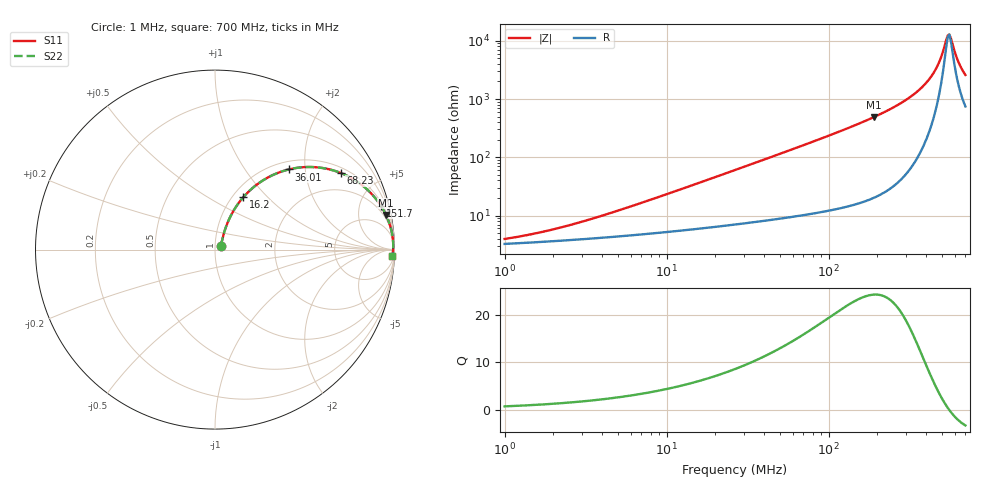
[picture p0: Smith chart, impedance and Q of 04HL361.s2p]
! Coilcraft 0402HL-361 Chip Inductor
! 20 July 2012
# MHz S MA R 50
!Freq  MagS11  AngS11  MagS21  AngS21  MagS12  AngS12  MagS22  AngS22
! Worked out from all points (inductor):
!   288 points, 1 MHz to 700 MHz, reference 50 ohm
!   read as one part in series: L = 360 nH near 6.21 MHz
!   highest Q = 24.2 at 190.6 MHz (marker M1), where L = 408 nH
!   self-resonance near 544.6 MHz
!   S11 on the Smith chart (normalised r, x): 1 MHz: 1.07, +0.05; 16.2 MHz: 1.12, +0.73; 36.01 MHz: 1.16, +1.64; 68.23 MHz: 1.20, +3.13; 151.7 MHz: 1.32, +7.42; 700 MHz: 16, -50
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1  0.03842 33.5  0.9682 -1.3  0.9682 -1.3  0.03842 33.5
1.690458  0.05023 45.2  0.9652 -2.1  0.9652 -2.1  0.05023 45.2
2.991129  0.07507 56.2  0.9603 -3.7  0.9603 -3.7  0.07507 56.2
8.946856  0.195 65.1  0.9347 -10.9  0.9347 -10.9  0.195 65.1
16.19625  0.3313 61.6  0.8917 -19.1  0.8917 -19.1  0.3313 61.6
26.7612  0.4964 53.8  0.8128 -29.5  0.8128 -29.5  0.4964 53.8
36.00623  0.6072 47.4  0.739 -37.2  0.739 -37.2  0.6072 47.4
49.56361  0.7226 39.5  0.6374 -46.1  0.6374 -46.1  0.7226 39.5
68.22573  0.82 31.4  0.5222 -54.9  0.5222 -54.9  0.82 31.4
80.04622  0.8593 27.6  0.4639 -59.1  0.4639 -59.1  0.8593 27.6
151.6741  0.9553 14.9  0.2573 -72.6  0.2573 -72.6  0.9553 14.9
190.5653  0.9719 11.4  0.1986 -76.2  0.1986 -76.2  0.9719 11.4
239.4286  0.9827 8.5  0.1475 -79.1  0.1475 -79.1  0.9827 8.5
329.5804  0.991 4.9  0.08592 -81.5  0.08592 -81.5  0.991 4.9
414.089  0.9932 2.7  0.04711 -80.4  0.04711 -80.4  0.9932 2.7
474.8682  0.9933 1.4  0.0254 -74.1  0.0254 -74.1  0.9933 1.4
508.5255  0.993 0.8  0.01534 -62.6  0.01534 -62.6  0.993 0.8
544.5684  0.9925 0.2  0.008032 -21.2  0.008032 -21.2  0.9925 0.2
557.1418  0.9923 -0.0  0.007745 4.9  0.007745 4.9  0.9923 -0.0
570.0054  0.992 -0.2  0.009027 27.8  0.009027 27.8  0.992 -0.2
624.4992  0.9907 -1.1  0.02068 62.8  0.02068 62.8  0.9907 -1.1
700  0.9884 -2.1  0.03816 71.2  0.03816 71.2  0.9884 -2.1
